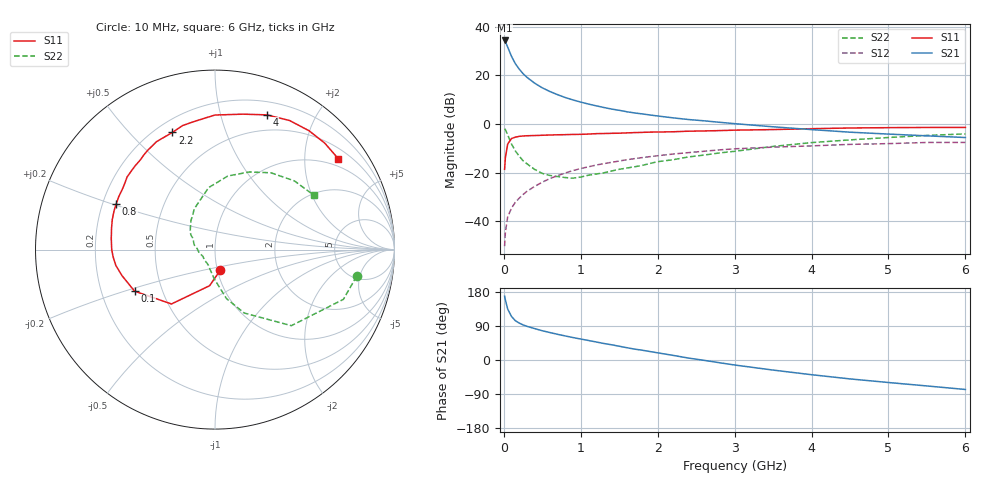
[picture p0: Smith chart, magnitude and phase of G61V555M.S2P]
! SIEMENS Small Signal Semiconductors
! BFG193
! Si NPN RF Bipolar Junction Transistor in SOT223
! VCE = 1.5 V  IC = 55 mA
! Common Emitter S-Parameters:  August  1996
# GHz  S  MA  R  50
!  f  S11  S21  S12  S22
! GHz  MAG  ANG  MAG  ANG  MAG  ANG  MAG  ANG
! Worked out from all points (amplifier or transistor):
!   36 points, 10 MHz to 6 GHz, reference 50 ohm
!   highest |S21| = 34.4 dB at 10 MHz (marker M1)
!   |S21| within 3 dB of that: start of sweep to 53.47 MHz
!   unconditionally stable (mu >= 1): start of sweep to 11.14 MHz; 262.9 MHz to 2.855 GHz
!   at 250 MHz: K = 0.99, MSG = 24.8 dB, |S12| = -28.9 dB
!   at 1.4 GHz: K = 1.09, MAG = 9.1 dB, |S12| = -15.7 dB
!   at 6 GHz: K = 0.98, MSG = 1.0 dB, |S12| = -7.5 dB
!   S11 on the Smith chart (normalised r, x): 10 MHz: 1.03, -0.24; 100 MHz: 0.35, -0.22; 800 MHz: 0.26, +0.21; 2.2 GHz: 0.26, +0.67; 4 GHz: 0.33, +1.40; 6 GHz: 0.77, +2.87
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0.01  0.1176 -75.0  52.23 168.4  0.0031 77.7  0.8033 -10.6
0.02  0.2034 -98.5  49.43 158.4  0.006 75.1  0.767 -21.2
0.05  0.3882 -128.7  38.12 134.4  0.0124 64.1  0.6004 -44.9
0.1  0.5046 -152.7  24.58 114.7  0.0188 62.2  0.3889 -65.3
0.15  0.5387 -164.5  17.37 103.6  0.0248 62.2  0.2805 -76.8
0.2  0.5594 -170.9  13.46 97.4  0.03 64.7  0.2193 -82.2
0.25  0.5688 -175.8  10.86 92.6  0.0357 65.8  0.1762 -88.7
0.3  0.5755 180.0  9.149 88.9  0.0415 66.6  0.1531 -93.3
0.4  0.5812 173.9  6.928 82.9  0.0524 67.0  0.1172 -102.8
0.5  0.589 168.1  5.553 77.2  0.064 66.4  0.0968 -111.2
0.6  0.5964 163.6  4.654 72.4  0.0761 65.5  0.0879 -120.0
0.8  0.6061 155.3  3.502 63.4  0.0991 61.9  0.0796 -141.7
1.1  0.6231 143.9  2.576 51.5  0.1325 56.1  0.089 -167.3
1.3  0.6398 136.7  2.191 43.6  0.1541 51.7  0.0997 176.5
1.6  0.6592 127.1  1.79 32.4  0.1851 44.7  0.1251 161.7
2.2  0.6946 110.0  1.342 12.2  0.2424 30.1  0.1852 137.7
2.8  0.734 94.6  1.089 -7.1  0.2948 15.5  0.255 116.9
3.5  0.7706 78.3  0.879 -26.6  0.336 -2.4  0.3473 95.9
4  0.804 69.0  0.77 -38.8  0.3562 -12.3  0.4162 80.1
4.5  0.8306 60.0  0.681 -49.9  0.3827 -22.4  0.4732 66.1
5.5  0.852 44.2  0.573 -68.5  0.419 -45.3  0.5849 40.9
6  0.8536 36.3  0.529 -77.8  0.4194 -58.4  0.6288 28.8
